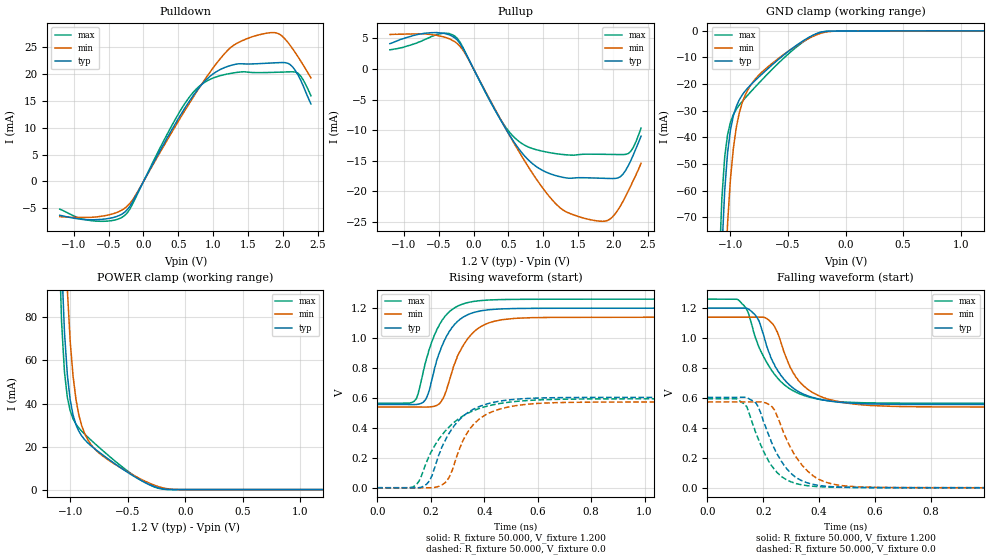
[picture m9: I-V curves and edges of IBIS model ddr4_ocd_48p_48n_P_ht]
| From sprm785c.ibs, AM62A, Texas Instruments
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|   Model ddr4_ocd_48p_48n_P_ht
[Model] ddr4_ocd_48p_48n_P_ht
Model_type I/O
Polarity   Non-Inverting
Enable   Active-High
Vinl =  0.700V
Vinh =  0.900V
Vmeas =  0.600V
C_comp   2.252pF   2.248pF   2.343pF
[Model Spec]
Vinh   0.900V   0.820V   0.980V
Vinl   0.700V   0.620V   0.780V
Vmeas   0.600V   NA   NA
[Temperature Range]   25.000   0.125k   -40.000
[Voltage Range]   1.200V   1.140V   1.260V
[Pullup Reference]   1.200V   1.140V   1.260V
[Pulldown Reference]   0.0V   0.0V   0.0V
[C Comp Corner]
C_comp   2.252pF   2.248pF   2.343pF
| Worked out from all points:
|   slope of the pulldown table from 0 to 0.18 V, typ, clamps not added: 41.3 ohm
|   slope of the pullup table from 0 to 0.18 V, typ, clamps not added: 45.2 ohm
|   GND clamp passes 1 mA (typ) near -0.25 V on its own axis
|   POWER clamp passes 1 mA (typ) near -0.25 V on its own axis
|   rising waveform, R_fixture 50.000, V_fixture 1.200: 20-80 % time 80.5ps typ, 89.8ps min, 80.2ps max; typ from 0.557 V to 1.2 V
|   rising waveform, R_fixture 50.000, V_fixture 0.0: 20-80 % time 113ps typ, 102ps min, 144ps max; typ from 0.002 V to 0.605 V
|   falling waveform, R_fixture 50.000, V_fixture 1.200: 20-80 % time 103ps typ, 104ps min, 113ps max; typ from 1.2 V to 0.557 V
|   falling waveform, R_fixture 50.000, V_fixture 0.0: 20-80 % time 93.6ps typ, 103ps min, 87.9ps max; typ from 0.605 V to 0.002 V
[Pulldown]
|Voltage   I(typ)   I(min)   I(max)
-1.2V     -6.264mA   -6.528mA   -5.12mA
-718mV    -7.094mA   -6.621mA   -7.306mA
-272mV    -5.718mA   -4.993mA   -6.333mA
-124mV    -3.019mA   -2.758mA   -3.321mA
359mV     8.521mA    8.102mA    9.244mA
656mV     14.86mA    14.47mA    15.63mA
953mV     19.51mA    20.27mA    18.93mA
1.324V    21.75mA    25.52mA    20.2mA
1.918V    22.03mA    27.5mA     20.26mA
2.14V     21.21mA    24.57mA    20.34mA
2.252V    18.83mA    22.38mA    19.58mA
2.4V      14.38mA    19.21mA    15.9mA
[Pullup]
|Voltage   I(typ)   I(min)   I(max)
-1.2V     4.136mA    5.634mA    3.131mA
-532mV    5.95mA     5.511mA    5.617mA
-346mV    5.576mA    4.926mA    5.781mA
-198mV    4.214mA    3.733mA    4.439mA
247mV     -5.43mA    -5.321mA   -5.505mA
544mV     -11.33mA   -11.44mA   -10.72mA
878mV     -15.78mA   -17.64mA   -13.13mA
1.324V    -17.8mA    -23.34mA   -14.03mA
1.955V    -17.9mA    -24.54mA   -13.96mA
2.103V    -17.61mA   -22.41mA   -13.99mA
2.252V    -15mA      -19.11mA   -13.47mA
2.4V      -10.99mA   -15.4mA    -9.668mA
[GND_clamp]
|Voltage   I(typ)   I(min)   I(max)
-1.2V     -396.3mA   -450.8mA   -370.5mA
-1.1V     -118.3mA   -172.8mA   -91.44mA
-1.075V   -83.02mA   -129.3mA   -63.08mA
-1.05V    -59.94mA   -96.19mA   -47.32mA
-1.025V   -45.76mA   -72.24mA   -38.96mA
-1V       -37.22mA   -55.56mA   -34.32mA
-975mV    -31.95mA   -44.18mA   -31.47mA
-925mV    -26.07mA   -31.12mA   -27.96mA
-775mV    -18.22mA   -17.64mA   -20.64mA
-425mV    -5.392mA   -5.54mA    -6.048mA
-175mV    -232.3uA   -493.9uA   -237.3uA
1.2V      0A         0A         0A
[POWER_clamp]
|Voltage   I(typ)   I(min)   I(max)
-1.2V     594.8mA    732.7mA    623.3mA
-1.1V     157.8mA    248.4mA    121.5mA
-1.075V   106.2mA    179.2mA    77.8mA
-1.05V    73.23mA    128.5mA    54.67mA
-1.025V   53.34mA    92.89mA    42.85mA
-1V       41.61mA    68.72mA    36.57mA
-975mV    34.56mA    52.6mA     32.87mA
-925mV    27.12mA    34.66mA    28.61mA
-825mV    20.64mA    21.33mA    23.28mA
-675mV    14.45mA    14mA       16.15mA
-200mV    388.1uA    876.1uA    237.4uA
1.2V      0A         0A         0A
[Ramp]
| variable   typ   min   max
dV/dt_r   0.362/0.113n   0.375/0.109n   0.356/0.145n
dV/dt_f   0.386/0.102n   0.391/0.110n   0.416/0.112n
R_load = 60.000
[Rising Waveform]
R_fixture= 50.000
V_fixture= 1.200
V_fixture_min= 1.140
V_fixture_max= 1.260
|time   V(typ)   V(min)   V(max)
0s        557.3mV    540.5mV    565.5mV
144ps     557.5mV    540.5mV    590.8mV
186ps     609.1mV    540.4mV    874.1mV
231ps     896.9mV    560.2mV    1.083V
256ps     1.001V     638.2mV    1.151V
288ps     1.09V      823.8mV    1.2V
366ps     1.173V     1.049V     1.246V
436ps     1.192V     1.112V     1.256V
576ps     1.198V     1.136V     1.259V
3ns       1.2V       1.14V      1.26V
[Rising Waveform]
R_fixture= 50.000
V_fixture= 0.0
V_fixture_min= 0.0
V_fixture_max= 0.0
|time   V(typ)   V(min)   V(max)
0s        1.757mV    1.962mV    3.04mV
140ps     1.699mV    1.952mV    14.84mV
197ps     53.29mV    2.105mV    224.9mV
241ps     270.2mV    20.35mV    352.1mV
268ps     363.7mV    68.76mV    406.8mV
317ps     473.4mV    304.9mV    477mV
357ps     523.7mV    419mV      514.2mV
487ps     587mV      539.5mV    571.5mV
827ps     604.8mV    573.5mV    594.9mV
3ns       605.2mV    574.6mV    595.8mV
[Falling Waveform]
R_fixture= 50.000
V_fixture= 1.200
V_fixture_min= 1.140
V_fixture_max= 1.260
|time   V(typ)   V(min)   V(max)
0s        1.2V       1.14V      1.26V
129ps     1.2V       1.14V      1.221V
147ps     1.194V     1.14V      1.167V
179ps     1.135V     1.14V      967.7mV
213ps     943.1mV    1.13V      836.1mV
249ps     792.2mV    1.047V     739.1mV
315ps     656.6mV    744.4mV    641.4mV
425ps     584.1mV    597.4mV    584.8mV
775ps     557.7mV    541.8mV    565.7mV
3ns       557.3mV    540.4mV    565.5mV
[Falling Waveform]
R_fixture= 50.000
V_fixture= 0.0
V_fixture_min= 0.0
V_fixture_max= 0.0
|time   V(typ)   V(min)   V(max)
0s        605.2mV    574.6mV    595.8mV
105ps     605.2mV    574.6mV    595mV
136ps     605.2mV    574.6mV    556mV
179ps     552.5mV    574.6mV    342.1mV
227ps     320.1mV    549.5mV    158.5mV
294ps     108.1mV    284.1mV    46.49mV
368ps     29.78mV    97.63mV    14.22mV
448ps     9.221mV    27.35mV    6.443mV
608ps     3.08mV     4.786mV    3.857mV
3ns       1.756mV    1.955mV    3.04mV
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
